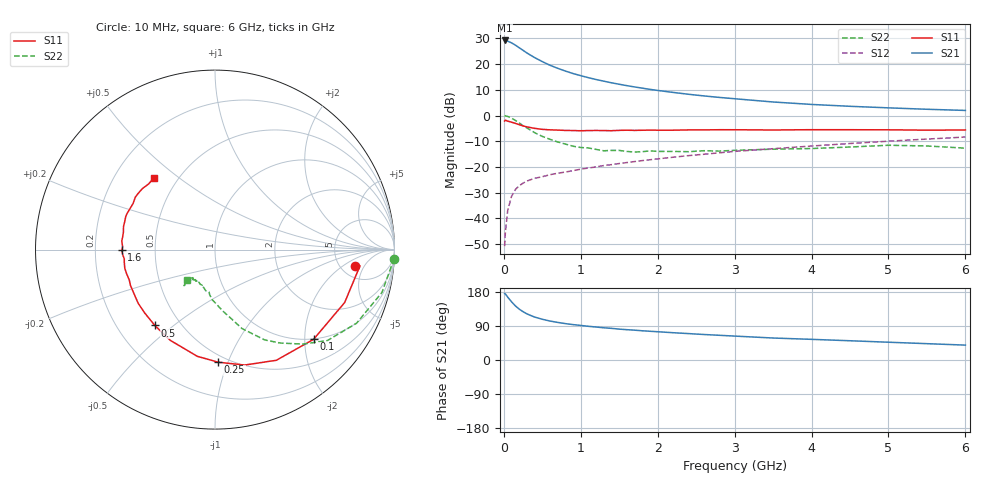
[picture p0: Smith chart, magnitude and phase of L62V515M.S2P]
!  INFINEON TECHNOLOGIES Small Signal Semiconductors
! BFR380L3 , Si-NPN RF-Transistor in TSLP-3-1
!  Vce=2.5 V,  Ic=15 mA
! Common Emitter S-Parameters:  07. March 2005
#  GHz  S  MA  R  50
! f  S11  S21  S12  S22
! GHz  Mag  Ang  Mag  Ang  Mag  Ang  Mag  Ang
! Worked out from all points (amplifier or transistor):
!   36 points, 10 MHz to 6 GHz, reference 50 ohm
!   highest |S21| = 29.2 dB at 10 MHz (marker M1)
!   |S21| within 3 dB of that: start of sweep to 208.2 MHz
!   unconditionally stable (mu >= 1): 1.961 GHz to 4.794 GHz
!   at 250 MHz: K = 0.32, MSG = 25.8 dB, |S12| = -26.3 dB
!   at 1.4 GHz: K = 0.93, MSG = 15.9 dB, |S12| = -19.1 dB
!   at 6 GHz: K = 0.97, MSG = 5.2 dB, |S12| = -8.3 dB
!   S11 on the Smith chart (normalised r, x): 10 MHz: 6.63, -3.23; 100 MHz: 0.99, -2.21; 250 MHz: 0.45, -0.92; 500 MHz: 0.36, -0.43; 1.6 GHz: 0.32, -0.00; 6 GHz: 0.37, +0.41
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0.01  0.7832 -6.9  28.76 175.3  0.0029 83.9  1.001 -2.9
0.02  0.8128 -6.4  28.7 174.4  0.0054 89.7  0.9844 -6.0
0.05  0.7803 -22.2  27.89 166.0  0.0142 80.3  0.9604 -14.4
0.1  0.7427 -42.3  25.81 153.6  0.0269 71.4  0.889 -27.5
0.15  0.705 -61.0  23.34 142.8  0.0365 62.9  0.8053 -39.0
0.2  0.6641 -75.6  20.75 134.2  0.0433 59.0  0.7187 -47.1
0.25  0.6274 -88.4  18.48 127.5  0.0486 54.8  0.6347 -55.1
0.3  0.6028 -99.4  16.42 121.7  0.0535 52.3  0.5742 -61.2
0.4  0.5635 -116.3  13.37 113.3  0.0603 50.0  0.465 -71.1
0.5  0.5395 -128.4  11.16 107.5  0.0648 49.5  0.3936 -76.9
0.6  0.5274 -138.0  9.476 102.8  0.0709 49.7  0.3455 -82.7
0.7  0.5222 -144.9  8.275 99.2  0.0758 50.7  0.3068 -88.0
0.9  0.5113 -157.2  6.544 93.4  0.085 52.8  0.2534 -96.7
1.1  0.5106 -164.7  5.436 88.9  0.0957 54.8  0.2348 -102.7
1.4  0.508 -174.1  4.324 83.5  0.1112 57.1  0.2104 -109.7
1.6  0.5194 -179.7  3.807 80.0  0.1222 58.2  0.2006 -117.6
2.2  0.5195 169.2  2.814 72.0  0.155 60.7  0.2009 -122.2
2.8  0.5303 159.7  2.252 65.2  0.1887 61.9  0.2039 -129.4
3.5  0.5237 150.6  1.834 58.0  0.227 61.2  0.2222 -129.8
4.5  0.5304 143.9  1.512 50.8  0.2864 60.7  0.2448 -130.4
5.5  0.5203 135.5  1.324 43.1  0.3491 57.9  0.2565 -130.9
6  0.5247 130.2  1.257 39.3  0.3824 56.0  0.2325 -132.8
